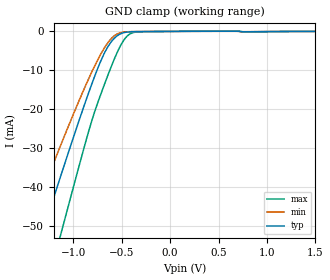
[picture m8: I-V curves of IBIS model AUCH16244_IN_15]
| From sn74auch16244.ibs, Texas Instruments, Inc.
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[Model]   AUCH16244_IN_15
Model_type  Input
Vinl=0.49
Vinh=1.04
| variable   typ   min   max
C_comp   3.45pF   2.71pF   4.07pF
[Temperature Range]   40   100   -40
| Ambient temperature   25   85   -40
[Voltage range]   1.5   1.4   1.6
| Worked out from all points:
|   GND clamp passes 1 mA (typ) near -0.54 V on its own axis
[GND Clamp]
| AUCH16244_IN_15
|   Voltage   I(typ)   I(min)   I(max)
-3.6V     -232.7mA   -194.4mA   -280.6mA
-1.51V    -66.74mA   -53.44mA   -87.74mA
-1.465V   -63.2mA    -50.52mA   -83.54mA
-1.33V    -52.64mA   -41.84mA   -70.92mA
-1.29V    -49.52mA   -39.29mA   -67.18mA
-1.13V    -37.18mA   -29.26mA   -52.22mA
-1.08V    -33.37mA   -26.18mA   -47.56mA
-815mV    -13.97mA   -10.77mA   -23.49mA
-695mV    -6.456mA   -4.934mA   -14.76mA
-575mV    -1.754mA   -1.113mA   -7.055mA
-430mV    -139.2uA   -76.73uA   -919.2uA
1.5V      189.6pA    534nA      87.79pA
